(* Logix 5000 AddOnInstructionDefinition export AMCI_5034_PTO_AM_MRP; software revision 37.00 *)

TYPE AMCI_5034_PTO_AM_Input_Data :
STRUCT
   ConnectionFaulted : DINT;
   MovingCW : BOOL;
   MovingCCW : BOOL;
   InHoldState : BOOL;
   Stopped : BOOL;
   AtHome : BOOL;
   Accelerating : BOOL;
   Decelerating : BOOL;
   MoveComplete : BOOL;
   HomeInvalid : BOOL;
   InvalidProfile : BOOL;
   PositionInvalid : BOOL;
   InputError : BOOL;
   CommandError : BOOL;
   ConfigurationError : BOOL;
   ModuleOK : BOOL;
   GeneralPurposeOutputStatus : BOOL;
   Input1Active : BOOL;
   Input2Active : BOOL;
   Input3Active : BOOL;
   Input4Active : BOOL;
   bit_20_reserved : BOOL;
   bit_21_reserved : BOOL;
   bit_22_reserved : BOOL;
   EncoderFollowerMode : BOOL;
   BlendMoveRunning : BOOL;
   BlendMoveAcknowledge : BOOL;
   MinimumRegistrationProgrammed : BOOL;
   EncoderMotionDirection : BOOL;
   MultipleInputsWithSameFunction : BOOL;
   FSCExceedsNumberOfDataBits : BOOL;
   AbsoluteEncoderSetupError : BOOL;
   bit_31_reserved : BOOL;
   CurrentPosition : DINT;
   EncoderPosition : DINT;
   CapturedPosition : DINT;
END_STRUCT
END_TYPE

TYPE AMCI_5034_PTO_AM_Output_Data :
STRUCT
   Command_Word : DINT;
   TargetPosition : DINT;
   TargetVelocity : UDINT;
   Acceleration : DINT;
   Deceleration : DINT;
END_STRUCT
END_TYPE

ADD_ON_INSTRUCTION AMCI_5034_PTO_AM_MRP   (* revision 1.0, vendor AMCI, ExecuteEnableInFalse *)
// AMCI Preset Position
// Revision note:
// 10/01/2025 Intial release
// Help:
// MOTION REDEFINE POSITION: Sets the Current Motor Position to the value in the Target Position field of the AOI.  This command will also reset the Position Invalid status bit.
// AXIS INPUT DATA:  Input data from the AMCI 5034-PTO-AM.   Uses the AMCI_5034_PTO_Input_Data User Defined Data Type.
// AXIS OUTPUT DATA; Output data from the AOI to the AMCI 5034-PTO-AM.    Uses the AMCI_5034_PTO_Output_Data User Defined Data Type.
// TARGET POSITION: Position to which the Motor Position is to be set.
// SAVE_IN_FLASH_0_NO_1_YES:   Saves the offset in the flash memory.    Only used on the SVXXXE2 units.  Must be zero on all other units.
// EN (Enable) Set when rung is true, Reset when rung is false
// DN (Done) Set when command is sent to the motion device.  Reset when the rung is false.
// ER (Error) Set when a command or input error failed to clear.  Reset when the rung is false.
VAR_IN_OUT
   Axis_Input_Data : AMCI_5034_PTO_AM_Input_Data; {required}
   Axis_Output_Data : AMCI_5034_PTO_AM_Output_Data; {required}
END_VAR
VAR_INPUT
   TargetPosition : DINT; {required}
END_VAR
VAR_OUTPUT
   EN : BOOL; {visible}   // set when rung with AOI is true
   DN : BOOL; {access Read Only, visible}   // set when preset motor position command sent to motion axis
   ER : BOOL; {access Read Only, visible}   // set when input, command, or configuraiton error
END_VAR
VAR
   command_data_block : DINT[5];
        [0]   // Command Bits MSW
        [1]   // Target Position
        [2]   // Upper Target Position
        [3]   // Lower Target Position
        [4]   // Upper Programmed Speed
END_VAR

ROUTINE EnableInFalse   (* ladder *)
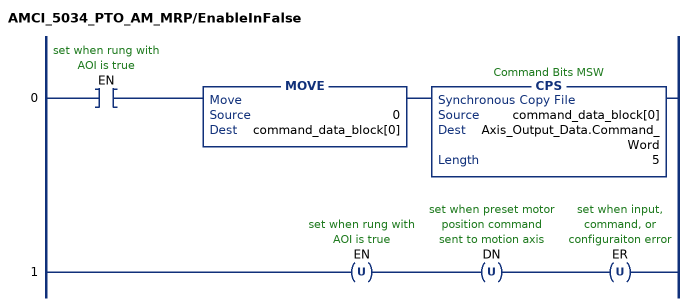
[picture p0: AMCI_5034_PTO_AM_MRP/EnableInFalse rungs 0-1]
   0: XIC(EN)MOVE(0,command_data_block[0])CPS(command_data_block[0],Axis_Output_Data.Command_Word,5);
   1: OTU(EN)OTU(DN)OTU(ER);
END_ROUTINE

ROUTINE Logic   (* ladder *)
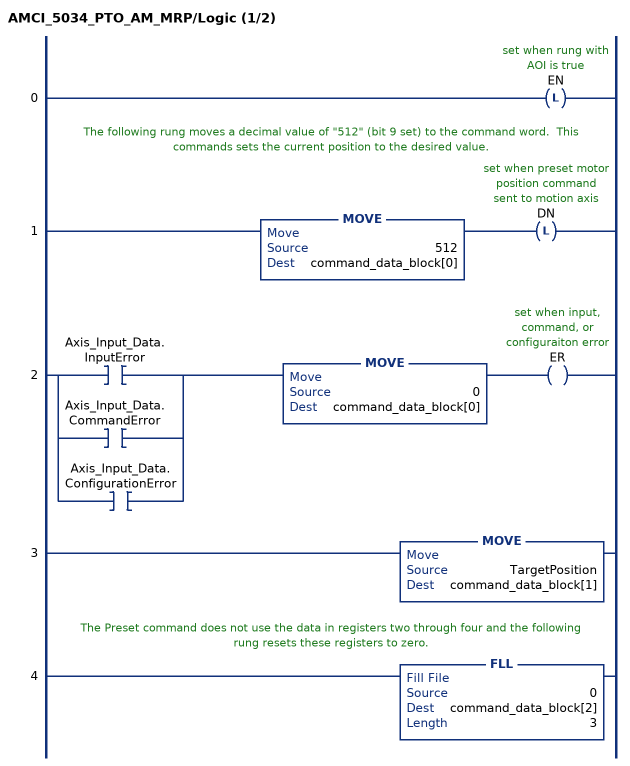
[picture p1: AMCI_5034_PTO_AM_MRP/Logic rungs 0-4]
   0: OTL(EN);
   // The following rung moves a decimal value of "512" (bit 9 set) to the command word.  This commands sets the current position to the desired value.
   1: MOVE(512,command_data_block[0])OTL(DN);
   2: [XIC(Axis_Input_Data.InputError) ,XIC(Axis_Input_Data.CommandError) ,XIC(Axis_Input_Data.ConfigurationError) ]MOVE(0,command_data_block[0])OTE(ER);
   3: MOVE(TargetPosition,command_data_block[1]);
   // The Preset command does not use the data in registers two through four and the following rung resets these registers to zero.
   4: FLL(0,command_data_block[2],3);
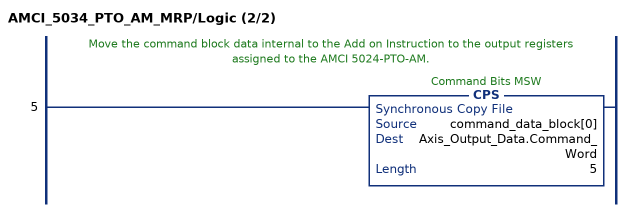
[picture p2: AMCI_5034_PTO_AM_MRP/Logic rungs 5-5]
   // Move the command block data internal to the Add on Instruction to the output registers assigned to the AMCI 5024-PTO-AM.
   5: CPS(command_data_block[0],Axis_Output_Data.Command_Word,5);
END_ROUTINE
END_ADD_ON_INSTRUCTION
